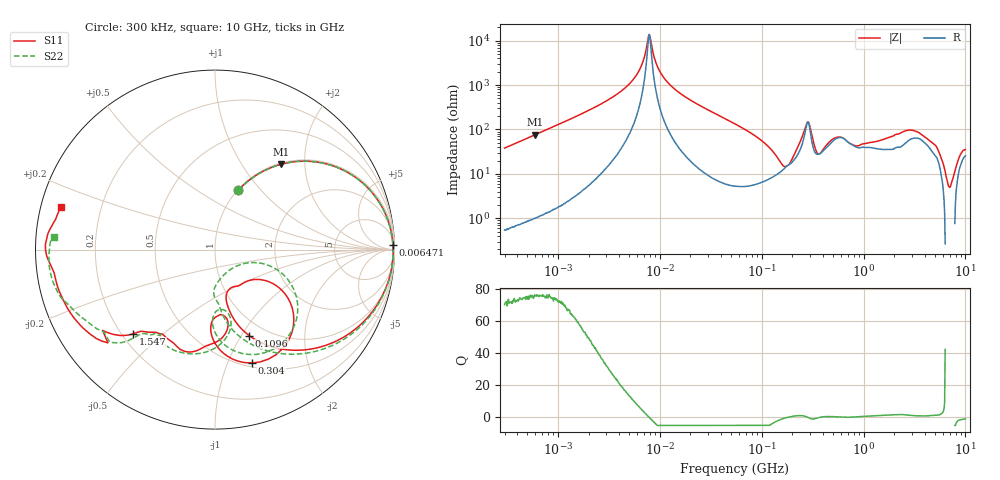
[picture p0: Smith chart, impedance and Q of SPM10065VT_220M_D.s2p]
! S-Parameter Data Generated by TDK Corporation
! Copyright(C) 2020 TDK Corporation.
! All Rights Reserved.
! TDK P/N: SPM10065VT-220M-D (Inductor)
! Property: L=22uH at 100kHz
! Size(LxWxT): 10.5x10x6.5mm
! Model Type: s2p (Touchstone File Format Version 1.0)
! Frequency: DC=Yes Start=0.3MHz Stop=10000MHz 802points Log-sweep
! Model Generated on Apr. 23, 2020
! Port Assignments:
!  1 ---@@@--- 2
! Applicable Conditions:
!  Temperature = 25 degC
!  DC Bias Current = 0 A
!  Small Signal Operation
! Terms and conditions regarding TDK Simulation Models
! (1)This simulation model is being provided solely for informational purposes. Please refer to the specifications of the products in terms of detailed characteristics of such products.
! (2)In no event shall TDK Corporation of any of its subsidiaries be liable for any loss or damage arising, directly or indirectly,
!  From any information contained in this simulation model, including, but not limited to loss or damages arising from any inaccuracies, omissions or errors in connection with such information.
! (3)Any and all copyrights on this simulation model are owned by TDK Corporation.
!  Duplication or redistribution of this simulation model without prior written permission from TDK Corporation is prohibited.
! (4)This simulation model is subject to any modification or change without any prior notice.
! (5)Neither TDK Corporation nor any of its subsidiaries shall make any warranty, express or implied,
!  Including but not limited to the correctness, implied warranties of merchantability and fitness for a particular purpose with respect to this simulation models.
! (6)The use of this simulation model shall be deemed to have consented to the terms and conditions hereof.
# Hz S MA R 50
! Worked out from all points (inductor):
!   801 points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, 300 kHz to 10 GHz, reference 50 ohm
!   read as one part in series: L = 20.2 uH near 318.3 kHz
!   highest Q = 75.8 at 601.5 kHz (marker M1), where L = 20.2 uH
!   self-resonance near 7.772 MHz
!   S11 on the Smith chart (normalised r, x): 300 kHz: 1.01, +0.76; 6.471 MHz: 26, +76; 109.6 MHz: 0.83, -1.08; 304 MHz: 0.54, -1.23; 1.547 GHz: 0.24, -0.40; 10 GHz: 0.06, +0.13
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300000  0.3557 68.5  0.9295 -20.7  0.9295 -20.8  0.3554 68.5
601544  0.6033 52.1  0.7899 -37.1  0.7898 -37.2  0.6032 52.1
1713600  0.9084 23.5  0.4021 -65.5  0.4019 -65.6  0.9086 23.4
4239428  0.9844 6.9  0.1315 -80.1  0.1315 -80.1  0.9844 6.8
6470506  0.992 1.4  0.04048 -78.7  0.04051 -78.7  0.9922 1.1
7890546  0.9927 -1.1  0.007196 -0.9  0.007191 -0.4  0.9928 -1.4
9671944  0.9916 -3.7  0.04176 75.9  0.04175 75.9  0.9917 -4.1
1.694973e7  0.9775 -12.0  0.1664 74.8  0.1664 74.8  0.9776 -12.7
5.477226e7  0.8041 -42.2  0.5648 44.5  0.5646 44.5  0.8035 -44.5
1.096398e8  0.5153 -68.3  0.8015 12.7  0.8012 12.7  0.5101 -73.6
2.102074e8  0.2487 -45.7  0.8044 -27.8  0.8041 -27.8  0.1402 -55.5
2.694285e8  0.5665 -39.4  0.4695 -50.1  0.4693 -50.1  0.4963 -27.2
3.040112e8  0.6649 -71.8  0.4503 -14.4  0.4501 -14.4  0.6378 -64.4
3.126428e8  0.6348 -78.3  0.5166 -14.3  0.5164 -14.3  0.6147 -72.0
3.601167e8  0.4493 -93.0  0.665 -31.1  0.6647 -31.1  0.4434 -90.9
4.568044e8  0.4357 -80.5  0.5887 -53.3  0.5884 -53.3  0.3551 -79.0
6.656121e8  0.5914 -106.2  0.4266 -61.7  0.4265 -61.7  0.5883 -99.6
9.330971e8  0.5567 -122.5  0.4263 -85.3  0.4261 -85.3  0.5611 -122.8
1.547353e9  0.6543 -134.2  0.2509 -135.6  0.2507 -135.7  0.651 -132.2
1.767019e9  0.7209 -138.6  0.1924 -151.3  0.1921 -151.2  0.7164 -134.3
3.387826e9  0.8874 -159.7  0.03622 -164.5  0.03626 -164.3  0.8723 -159.2
1e10  0.8904 164.7  0.02449 137.1  0.02442 137.3  0.9011 175.5
